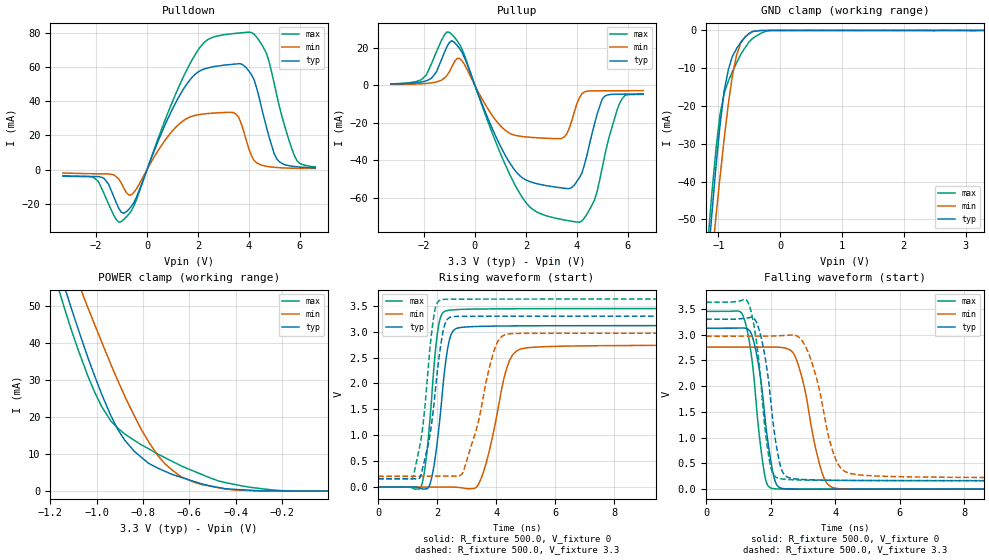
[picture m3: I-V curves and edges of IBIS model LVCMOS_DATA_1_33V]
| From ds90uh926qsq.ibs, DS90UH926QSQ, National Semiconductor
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[Model] LVCMOS_DATA_1_33V
Model_type 3-state
Enable Active-High
Vmeas = 1.65V
Cref = 0.0pF
Rref = 1.0e10
Vref = 0.0V
C_comp   2.75pF   2.32pF   3.18pF
[Voltage Range]   3.3V   2.97V   3.63V
[Temperature Range]   25.0   130.0   -40.0
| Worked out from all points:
|   slope of the pulldown table from 0 to 0.495 V, typ, clamps not added: 26.3 ohm
|   slope of the pullup table from 0 to 0.495 V, typ, clamps not added: 28.9 ohm
|   GND clamp passes 1 mA (typ) near -0.52 V on its own axis
|   POWER clamp passes 1 mA (typ) near -0.48 V on its own axis
|   rising waveform, R_fixture 500.0, V_fixture 0: 20-80 % time 359ps typ, 607ps min, 308ps max; typ from 0 V to 3.12 V
|   falling waveform, R_fixture 500.0, V_fixture 0: 20-80 % time 384ps typ, 534ps min, 352ps max; typ from 3.13 V to 0 V
|   rising waveform, R_fixture 500.0, V_fixture 3.3: 20-80 % time 418ps typ, 687ps min, 369ps max; typ from 0.159 V to 3.3 V
|   falling waveform, R_fixture 500.0, V_fixture 3.3: 20-80 % time 396ps typ, 612ps min, 345ps max; typ from 3.3 V to 0.162 V
[GND Clamp]
-3.3V     -551.2mA   -486.4mA   -587.6mA
-1.169V   -61.14mA   -71.51mA   -55.66mA
-1.109V   -48.96mA   -60.9mA    -43.45mA
-1.039V   -35.64mA   -48.93mA   -31.12mA
-978.3mV  -25.55mA   -39.39mA   -22.64mA
-907.9mV  -15.99mA   -28.64mA   -16.63mA
-837.6mV  -10.21mA   -19.13mA   -13.29mA
-706.9mV  -4.789mA   -6.49mA    -8.554mA
-636.5mV  -3.113mA   -3.224mA   -6.259mA
-445.6mV  -245.1uA   -327.8uA   -2.09mA
-174.2mV  -754.2nA   1.165uA    -24.13uA
3.293V    2.005uA    0A         9.291uA
[POWER Clamp]
-3.3V     548.4mA    487.4mA    581.3mA
-1.169V   61.16mA    71.7mA     55.48mA
-1.139V   55.16mA    66.5mA     49.36mA
-1.109V   49.22mA    61.29mA    43.38mA
-1.079V   43.51mA    56.1mA     37.91mA
-1.039V   36.1mA     49.55mA    31.09mA
-978.3mV  26.06mA    40.2mA     22.73mA
-907.9mV  16.45mA    29.64mA    16.89mA
-777.3mV  7.486mA    13.36mA    11.41mA
-676.8mV  4.488mA    5.724mA    8.051mA
-445.6mV  574.8uA    517.9uA    2.244mA
-3.35mV   -557.2nA   -7.985uA   426nA
[Pullup]
-3.3V     799.7uA    508.2uA    855.9uA
-1.702V   3.919mA    1.385mA    11.67mA
-1.008V   22.85mA    7.191mA    28.44mA
-606.4mV  19.72mA    14.48mA    21.99mA
790.7mV   -26.41mA   -18.14mA   -29.32mA
1.695V    -47.33mA   -26.93mA   -56.19mA
3.494V    -54.86mA   -27.57mA   -71.78mA
4.097V    -49.24mA   -6.649mA   -73mA
4.69V     -20.54mA   -2.871mA   -61.08mA
4.992V    -7.23mA    -2.848mA   -44.02mA
5.695V    -4.66mA    -2.813mA   -8.911mA
6.6V      -4.543mA   -2.795mA   -4.76mA
[Pulldown]
-3.3V     -3.683mA   -2.031mA   -3.933mA
-1.702V   -4.976mA   -2.544mA   -13.59mA
-1.008V   -24.97mA   -7.891mA   -30.41mA
-606.4mV  -21.35mA   -14.67mA   -23.89mA
891.2mV   32.16mA    20.78mA    35.92mA
1.997V    57.07mA    32.07mA    69.83mA
3.494V    61.82mA    32.43mA    79.78mA
3.997V    57.63mA    12mA       80.49mA
4.69V     24.52mA    1.886mA    67.83mA
5.092V    6.155mA    1.204mA    43.4mA
5.896V    1.587mA    710.6uA    4.788mA
6.6V      1.07mA     678.8uA    1.574mA
[Rising Waveform]
R_fixture=500.0
V_fixture=0
V_fixture_min=0
V_fixture_max=0
0s        24.71nV    508.9nV    71.69nV
1.45ns    -28.47mV   498nV      -5.636mV
1.6ns     -37.64mV   128.7nV    433.5mV
1.75ns    46.69mV    -1.228uV   1.283V
2.05ns    1.115V     -1.003uV   3.139V
2.4ns     2.816V     51.84uV    3.415V
3.4ns     3.102V     60.61mV    3.438V
4.4ns     3.111V     2.372V     3.443V
5.05ns    3.113V     2.689V     3.444V
49.98ns   3.12V      2.747V     3.448V
[Falling Waveform]
R_fixture=500.0
V_fixture=0
V_fixture_min=0
V_fixture_max=0
0s        3.126V     2.759V     3.452V
1.1ns     3.131V     2.759V     3.423V
1.4ns     3.02V      2.759V     2.611V
1.6ns     2.499V     2.759V     1.325V
1.8ns     1.523V     2.759V     322mV
2.1ns     229.6mV    2.76V      8.74mV
2.75ns    1.642mV    2.588V     751.4uV
3.6ns     563.4uV    302.3mV    352.2uV
4.1ns     390uV      10.77mV    248.8uV
49.98ns   5.177uV    13.54uV    3.307uV
[Rising Waveform]
R_fixture=500.0
V_fixture=3.3
V_fixture_min=2.97
V_fixture_max=3.63
0s        159mV      207.3mV    162.5mV
1.2ns     159mV      207.3mV    225.1mV
1.45ns    233.4mV    207.3mV    913.4mV
1.7ns     830.7mV    207.3mV    2.375V
1.9ns     1.663V     207.3mV    3.364V
2.2ns     3.02V      207.3mV    3.623V
2.85ns    3.297V     259.9mV    3.629V
3.95ns    3.299V     2.679V     3.63V
4.45ns    3.3V       2.959V     3.63V
49.98ns   3.3V       2.97V      3.63V
[Falling Waveform]
R_fixture=500.0
V_fixture=3.3
V_fixture_min=2.97
V_fixture_max=3.63
0s        3.3V       2.97V      3.63V
1.25ns    3.321V     2.97V      3.674V
1.55ns    3.254V     2.97V      2.908V
2ns       1.726V     2.972V     427.3mV
2.2ns     756.3mV    2.977V     220.8mV
2.4ns     301.2mV    2.983V     193.7mV
3.05ns    186.4mV    2.805V     175.9mV
4ns       172.4mV    602.7mV    169.6mV
4.75ns    168.4mV    277mV      167.8mV
49.98ns   161.7mV    215.3mV    164.5mV
[Ramp]
R_load = 500.0
dV/dt_r   1.872183E0/4E-10   1.647951E0/6.5E-10   2.068763E0/3E-10
dV/dt_f   1.882978E0/4E-10   1.652832E0/6.5E-10   2.079314E0/3.5E-10
